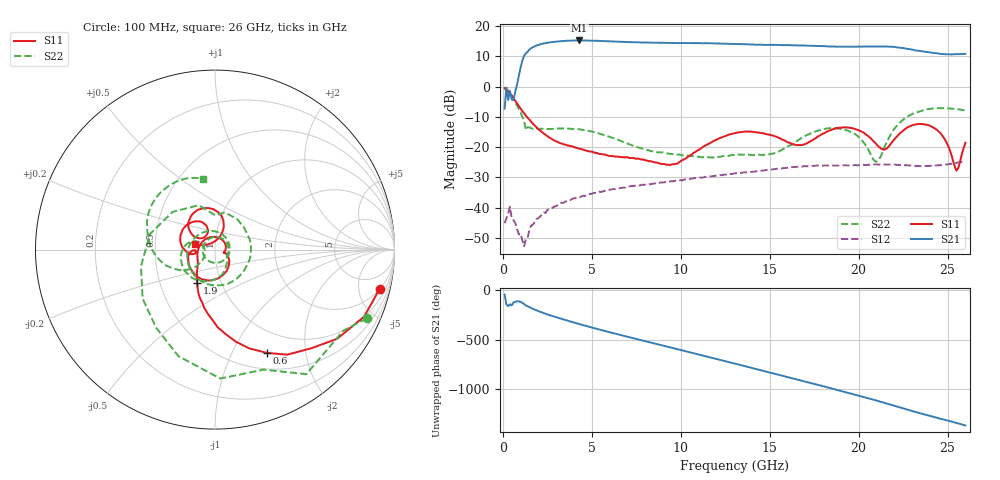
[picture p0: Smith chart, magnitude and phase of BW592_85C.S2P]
!Keysight Technologies,N5247A,US51370447,A.10.64.09
!Date: Thursday, March 05, 2020 07:08:28
!Correction: S11(Full 2 Port with power(1,2))
!S21(Full 2 Port with power(1,2))
!S12(Full 2 Port with power(1,2))
!S22(Full 2 Port with power(1,2))
!S2P File: Measurements: S11, S21, S12, S22:
# Hz S  dB  R 50
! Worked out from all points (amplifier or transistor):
!   260 points, 100 MHz to 26 GHz, reference 50 ohm
!   highest |S21| = 15.2 dB at 4.3 GHz (marker M1)
!   |S21| within 3 dB of that: 1.498 GHz to 22.98 GHz (21.49 GHz wide, 176 % of centre)
!   unconditionally stable (mu >= 1): start of sweep to end of sweep
!   at 4.4 GHz: K = 5.51, MAG = 15.4 dB, |S12| = -36.4 dB
!   at 13.1 GHz: K = 2.67, MAG = 14.2 dB, |S12| = -28.6 dB
!   at 26 GHz: K = 2.14, MAG = 11.7 dB, |S12| = -24.7 dB
!   S11 on the Smith chart (normalised r, x): 100 MHz: 2.03, -8.02; 600 MHz: 0.70, -1.37; 1.9 GHz: 0.77, -0.30; 26 GHz: 0.79, +0.05
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1e8  -0.51 -13.4  -7.31 -44.7  -45.14 7.5  -0.65 -24.4
6e8  -3.84 -63.5  -4.49 -124.5  -44.18 -28.8  -4.05 -109.0
1.2e9  -8.87 -96.3  10.26 -141.4  -52.74 4.2  -11.60 110.1
1.9e9  -13.52 -118.2  13.58 155.2  -43.78 13.8  -13.86 7.7
3e9  -18.12 -141.0  14.83 86.5  -39.49 -17.5  -13.95 -50.0
4.3e9  -20.51 -178.9  15.22 17.3  -36.74 -57.1  -14.14 -103.6
4.5e9  -20.86 173.0  15.22 7.2  -36.09 -65.2  -14.31 -112.2
5.6e9  -22.38 121.1  15.01 -46.3  -34.66 -100.1  -15.85 -163.2
6.5e9  -23.20 73.7  14.81 -87.9  -33.65 -130.6  -17.72 149.6
7.8e9  -24.14 15.1  14.56 -146.4  -32.46 -177.3  -20.42 68.1
8.8e9  -25.41 -13.8  14.45 169.0  -31.82 145.1  -21.70 -3.4
1.08e10  -21.72 -29.1  14.33 79.7  -30.21 65.6  -23.02 -149.8
1.2e10  -17.57 -59.4  14.24 25.1  -29.41 15.6  -23.32 118.5
1.31e10  -15.32 -96.3  14.05 -24.8  -28.64 -31.3  -22.54 45.7
1.5e10  -15.95 -159.9  13.78 -110.8  -27.48 -109.0  -22.37 -28.4
1.62e10  -18.80 -178.4  13.62 -166.5  -26.67 -158.0  -19.35 -55.1
1.74e10  -17.75 -168.9  13.47 137.8  -26.23 151.9  -15.24 -96.1
1.86e10  -14.03 166.5  13.21 81.3  -26.11 100.6  -13.70 -145.1
2e10  -14.44 123.6  13.20 15.1  -26.00 40.2  -16.67 164.3
2.17e10  -19.74 142.4  13.14 -71.8  -25.80 -43.2  -16.99 -138.4
2.36e10  -12.42 106.0  11.61 -170.7  -26.32 -139.4  -7.93 160.5
2.6e10  -18.57 165.0  10.80 73.4  -24.68 107.3  -7.94 99.8
